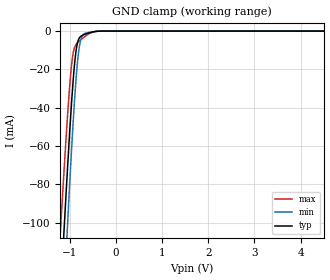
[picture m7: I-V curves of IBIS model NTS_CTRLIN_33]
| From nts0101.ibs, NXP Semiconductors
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|   Model NTS_CTRLIN_33
[Model]   NTS_CTRLIN_33
Model_type   Input
Vinh  =  2.145 | 0.65*Vcc
Vinl  =  1.155 | 0.35*Vcc
C_comp   0.6805pF   0.5009pF   1.0028pF
[Model Spec]
| Note: The input and output voltage ratings may be exceeded if the input and
|   output current ratings are observed (please refer to the data sheet)
|   Subparameter   typ   min   max
Vinh   2.145   1.950   2.340
Vinl   1.155   1.050   1.260
| Overshoot
S_overshoot_high   6.5   6.5   6.5   | Static overshoot
S_overshoot_low   -0.5   -0.5   -0.5
D_overshoot_high   7.2   7.2   7.2   | Dynamic overshoot
D_overshoot_low   -1.0   -1.0   -1.0
D_overshoot_time   3n   3n   3n
|Ambient temperature:   25   85   -40
[Temperature Range]   40   100   -25
[Voltage Range]   3.3   3.0   3.6
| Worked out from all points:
|   GND clamp passes 1 mA (typ) near -0.58 V on its own axis
|Process Range   nominal   slow   fast
[GND_clamp]
|   voltage   I(typ)   I(min)   I(max)
-3V       -1.012A    -1.143A    -900.6mA
-1.2V     -138.9mA   -176.6mA   -104.2mA
-1.12V    -103mA     -136.7mA   -71.92mA
-1.06V    -77.14mA   -107.7mA   -49.04mA
-1.04V    -68.78mA   -98.29mA   -41.85mA
-960mV    -37.6mA    -62.23mA   -17.76mA
-880mV    -13.76mA   -30.86mA   -7.69mA
-820mV    -5.176mA   -13.55mA   -5.806mA
-780mV    -3.231mA   -6.594mA   -4.942mA
-680mV    -1.752mA   -1.375mA   -3.069mA
-340mV    -20.37uA   -28.22uA   -16.89uA
5.5V      0A         0A         0A
